// TwinCAT 3 PLC project mongodbDataSave
// ProgramVersion: 3.1.4023.0
// libraries:
//   Tc2_Standard, * (Beckhoff Automation GmbH)
//   Tc2_System, * (Beckhoff Automation GmbH)
//   Tc2_Utilities, * (Beckhoff Automation GmbH)
//   Tc3_Database, * (Beckhoff Automation GmbH)
//   Tc3_JsonXml, * (Beckhoff Automation GmbH)
//   Tc3_Module, * (Beckhoff Automation GmbH)
// project tree:
//   DUTs/ demoDUT.TcDUT, eMyDbState.TcDUT
//   / PlcTask.TcTTO
//   POUs/ demoDataGen.TcPOU, JsonObjV5.TcPOU, MAIN.TcPOU
// (motion and I/O tree: see PLC project mongodb)
// real-time tasks:
//   TASK PlcTask: cycle T#10ms, priority 20, ADS port 350
//   TASK PlcTask1: cycle T#10ms, priority 21, ADS port 351

CONFIGURATION mongodbDataSave
    RESOURCE PLC ON TwinCAT3
        TASK PlcTask(INTERVAL := T#10ms, PRIORITY := 21);
        PROGRAM MAIN WITH PlcTask : MAIN;
        PROGRAM demoDataGen WITH PlcTask : demoDataGen;
    END_RESOURCE
END_CONFIGURATION

// ---- DUTs/demoDUT.TcDUT
TYPE demoDUT :
STRUCT
	timedata:TIMESTRUCT;
	realdata:REAL;
	eventdiscription:STRING;
END_STRUCT
END_TYPE

// ---- DUTs/eMyDbState.TcDUT
{attribute 'qualified_only'}
{attribute 'strict'}
TYPE eMyDbState :
(
	aggregation := 0,
	error := 10,
	idle := 20,
	readstruct := 30,
	validationissues := 40,
	validationremaining := 50,
	write := 60,
	createcollection := 70,
	dropcollection := 80,
	updateone := 90,
	updatemany := 100,
	writemany := 110,
	delete := 120,
	deletemany := 130
);
END_TYPE

// ---- POUs/MAIN.TcPOU
PROGRAM MAIN
VAR
	// 信号发生器
	ton1:Tc2_Standard.TON;
	// Json功能块
	jsonobj:JsonObjV5;
	// 时间采集
	gettime:Tc2_Utilities.NT_GetTime;
	
	// 数据库功能块
	fbNoSQLQueryBuilder_DocumentDB: FB_NoSQLQueryBuilder_DocumentDB;
	// 数据库请求命令
	fbNoSqlQuery : FB_NoSQLQueryEvt(sNetID := '', tTimeout := T#5S);
	// 数据库返回值
	fbNoSqlResult : FB_NoSQLResultEvt(sNetID := '', tTimeout := T#5S);
	// 数据插入
	InsertQueryOptions : Tc3_Database.T_QueryOptionDocumentDB_Insert;
	// 数据查询
	FindQueryOptions : Tc3_Database.T_QueryOptionDocumentDB_Find;
	// 数据查找
	datasearch : STRING(1000) := '{eventdiscription : "too large"}';
	// 查询返回，默认返回20个数据
	dataDocument : ARRAY[1..20] OF STRING(1000);
	// 返回信息
	InfoResult: Tc3_Database.I_TcMessage;
	
	// 数据
	demodata:demoDUT;
	// 转化的json对象
	jsondata:STRING(1000);
	// 查询异常数据
	read:BOOL;
END_VAR

// 调用信号发生器
SigGen();
// 读取系统时间
fbgettime();
// 数据赋值
setData();
// 结构体转化为json字符串
jsondata:=jsonobj.ObjToJsonStr(nData:= SIZEOF(demodata), pData:= ADR(demodata));
// 信号触发之后保存数据
IF ton1.Q THEN
	SaveData();
END_IF
// 查询
IF read THEN
	ReadData();
END_IF

ACTION fbgettime:
gettime(
	NETID:= '', 
	START:= ton1.Q, 
	TMOUT:= , 
	BUSY=> , 
	ERR=> , 
	ERRID=> , 
	TIMESTR=> demodata.timedata);
END_ACTION

ACTION ReadData:
FindQueryOptions.pFilter:= ADR(datasearch);
FindQueryOptions.cbFilter:= SIZEOF(datasearch); 

fbNoSQLQueryBuilder_DocumentDB.eQueryType := Tc3_Database.E_DocumentDbQueryType.Find;
fbNoSQLQueryBuilder_DocumentDB.sCollectionName := 'twincat';
fbNoSQLQueryBuilder_DocumentDB.pQueryOptions := ADR(FindQueryOptions);
fbNoSQLQueryBuilder_DocumentDB.cbQueryOptions := SIZEOF(FindQueryOptions);

IF fbNoSqlQuery.ExecuteDataReturn(hDBID:= 2, iNoSQLQueryBuilder:= fbNoSQLQueryBuilder_DocumentDB, pNoSQLResult:= ADR(fbNoSqlResult)) THEN
	IF fbNoSqlQuery.bError THEN
		InfoResult := fbNoSqlQuery.ipTcResult;
	ELSE
		IF fbNoSqlResult.ReadAsString(nStartIndex:= 0, nRecordCount:= 20, pData:= ADR(dataDocument), cbData:= SIZEOF(dataDocument), 
			MaxDocumentSize:= SIZEOF(dataDocument[1]), bDataRelease:= TRUE) THEN
			IF fbNoSqlResult.bError THEN
				InfoResult := fbNoSqlResult.ipTcResult;
			END_IF
		END_IF
	END_IF
END_IF
END_ACTION

ACTION SaveData:
InsertQueryOptions.pDocuments:= ADR(jsondata); 
InsertQueryOptions.cbDocuments:= SIZEOF(jsondata);

fbNoSQLQueryBuilder_DocumentDB.eQueryType := E_DocumentDbQueryType.InsertOne;
fbNoSQLQueryBuilder_DocumentDB.sCollectionName := 'twincat';
fbNoSQLQueryBuilder_DocumentDB.pQueryOptions := ADR(InsertQueryOptions);
fbNoSQLQueryBuilder_DocumentDB.cbQueryOptions := SIZEOF(InsertQueryOptions);

IF fbNoSQLQuery.Execute(2, fbNoSQLQueryBuilder_DocumentDB) THEN
	IF fbNoSQLQuery.bError THEN
		InfoResult := fbNoSQLQuery.ipTcResult;
	END_IF
END_IF
END_ACTION

ACTION setData:
// 采样记录的时间
demodata.timedata:=gettime.TIMESTR;
// 采样数据
demodata.realdata:=demoDataGen.dataout;
// 判断数据是否异常，加入描述
IF (demodata.realdata > 0.7) THEN
	demodata.eventdiscription:='too large';
ELSE
	demodata.eventdiscription:='normal state';
END_IF
END_ACTION

ACTION SigGen:
// 采样信号发生器
ton1(IN:= NOT ton1.Q, PT:= t#3s, Q=> , ET=> );
END_ACTION

END_PROGRAM

// ---- POUs/JsonObjV5.TcPOU
FUNCTION_BLOCK JsonObjV5
VAR_INPUT
END_VAR
VAR_OUTPUT
END_VAR
VAR
	// json功能块
	fbJsonRWDT : FB_JsonReadWriteDataType;
	fbJsonW : FB_JsonSaxWriter;
	fbJsonDP : FB_JsonDomParser;
	// 保存出的json字符串
	jsonStr : STRING(255);
	// json键值对地址
	ArrAdr : INT;
	// 键数组
	keyArr : ARRAY[0..999] OF STRING;
	// 值数组
	dataArr : ARRAY[0..999] OF STRING(255);
	// 值数据类型-未启用
	typeArr : ARRAY[0..999] OF STRING;
END_VAR

(*
* 功能 1 输入键（字符串）-值（任意数据类型）自动载入json
* 功能 2 输入键（字符串）自动返回值（任意数据类型，包括自定义数据类型以及JSON）
* 功能 3 JSON数据重置
* 功能 4 输出JSON字符串
* 功能 5 输入JSON字符串，转化为Json对象
* 功能 6 输入特定结构体对象，直接转化为Json字符串并返回
* 功能 7 输入JSON字符串，转化为结构体
*)

METHOD AddKeyValue : BOOL
VAR_INPUT
	key : STRING;// JSON键
 	nData : UDINT;// 值变量长度
 	pData : PVOID;// 值变量起始地址
END_VAR
VAR
	typestr : STRING;// 值变量数据类型
	tempstr : STRING;// 临时字符串变量
	keystr : STRING;// 键临时变量
END_VAR
(*
* 功能 1 输入键（字符串）-值（任意数据类型）自动载入json
*)
// 获得值变量的数据类型
typestr := fbJsonRWDT.GetDatatypeNameByAddress(nData := nData, pData := pData);
// 重置Json缓存
fbJsonW.ResetDocument();
// 添加数据到Json缓存
fbJsonRWDT.AddJsonValueFromSymbol(fbJsonW, typestr, nData, pData);
// 将当前缓存转为字符串
tempstr := fbJsonW.GetDocument();
// 将键转换为键格式
keystr := concat('"', concat(key, '"'));
// 写入数组缓存
keyArr[ArrAdr] := keystr;
dataArr[ArrAdr] := tempstr;
typeArr[ArrAdr] := typestr;
// 地址+1
ArrAdr := ArrAdr + 1;
END_METHOD

METHOD GetJsonStr : string(1000)
VAR_INPUT
END_VAR
VAR
	i: INT;
END_VAR
(*
* 功能 4 输出JSON字符串
*)
// 起始大括号
GetJsonStr := Tc2_Standard.CONCAT(GetJsonStr, '{');
// 遍历数据数组
FOR i := 0 TO ArrAdr - 1 BY 1 DO
	// 第二个元素开始要加上逗号分隔
	IF i > 0 THEN
		GetJsonStr := Tc2_Standard.CONCAT(GetJsonStr, ',');
	END_IF
	// 拼接键
	GetJsonStr := Tc2_Standard.CONCAT(GetJsonStr, KeyArr[i]);
	// 冒号分隔
	GetJsonStr := Tc2_Standard.CONCAT(GetJsonStr, ':');
	// 拼接值
	GetJsonStr := Tc2_Standard.CONCAT(GetJsonStr, dataArr[i]);
END_FOR
// 末尾大括号
GetJsonStr := Tc2_Standard.CONCAT(GetJsonStr, '}');
END_METHOD

METHOD GetKeyValue : BOOL
VAR_INPUT
	key : STRING;// JSON键
 	nData : UDINT;// 值变量返回长度
 	pData : PVOID;// 值变量返回起始地址
END_VAR
VAR
	typestr : STRING;// 值变量数据类型
	i : INT;// 键值
	sJson : string(255);
END_VAR
(*
* 功能 2 输入键（字符串）自动返回值（任意数据类型，包括自定义数据类型以及JSON）
*)
// Json中是否存在数据
IF arradr > 0 THEN
	// 获得值变量的数据类型
	typestr := fbJsonRWDT.GetDatatypeNameByAddress(nData := nData, pData := pData);
	// 遍历查找键值
	FOR i := 0 TO ArrAdr - 1 BY 1 DO
		// 给key拼接上""，判断键是否相等
		IF keyarr[i] = concat('"', concat(key, '"')) THEN
			// 如果相等，则返回值
			fbJsonRWDT.SetSymbolFromJson(sJson:= dataarr[i], sDatatype:= typestr, nData := nData, pData := pData);
			EXIT;
		END_IF
	END_FOR
END_IF
END_METHOD

METHOD JsonStrToObj : bool
VAR_INPUT
	JsonStr: STRING(1000);
	nData: UDINT;
	pData: PVOID;
END_VAR
VAR
	typestr: STRING;
END_VAR
(*
* 功能 7 输入JSON字符串，转化为结构体
*)
// 获得值变量的数据类型
typestr := fbJsonRWDT.GetDatatypeNameByAddress(nData := nData, pData := pData);
// 重置Json缓存
fbJsonW.ResetDocument();
// 将JSON字符串的信息写入特定数据
fbJsonRWDT.SetSymbolFromJson(sJson:= JsonStr, sDatatype:= typestr, nData:= nData, pData:= pData);
END_METHOD

METHOD ObjToJsonStr : STRING(1000)
VAR_INPUT
	nData: UDINT;
	pData: PVOID;
END_VAR
VAR
	typestr: STRING;
END_VAR
(*
* 功能 6 输入特定结构体对象，直接转化为Json字符串并返回
*)
// 获得值变量的数据类型
typestr := fbJsonRWDT.GetDatatypeNameByAddress(nData := nData, pData := pData);
// 重置Json缓存
fbJsonW.ResetDocument();
// 添加数据到Json缓存
fbJsonRWDT.AddJsonValueFromSymbol(fbJsonW, typestr, nData, pData);
// 将当前缓存转为字符串
fbJsonW.CopyDocument(pDoc:= ObjToJsonStr, nDoc:= SIZEOF(ObjToJsonStr));
END_METHOD

METHOD ResetObj : BOOL
VAR_INPUT
END_VAR
(*
* 功能 3 JSON数据重置
*)
// json键值对地址重置为0
ArrAdr := 0;
END_METHOD

END_FUNCTION_BLOCK

// ---- POUs/demoDataGen.TcPOU
PROGRAM demoDataGen
VAR
	t:REAL;
	dataout:REAL;
END_VAR

// 模拟信号发生器
t:=t+0.1;
IF t > 100 THEN
	t:=0;
END_IF
dataout:=SIN(t);

END_PROGRAM
